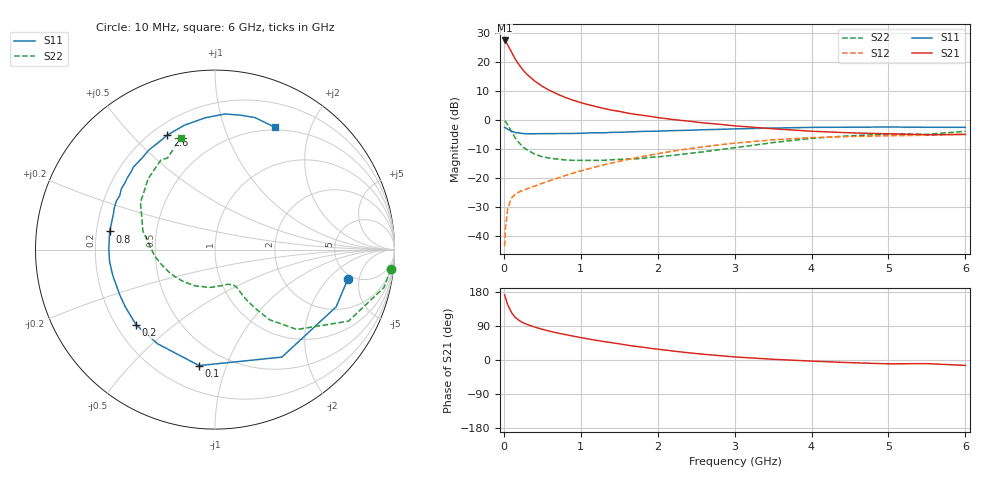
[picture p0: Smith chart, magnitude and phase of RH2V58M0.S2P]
! SIEMENS Small Signal Semiconductors
! BFR106
! Si NPN RF Bipolar Junction Transistor in SOT23
! VCE = 2.5 V  IC = 8 mA
! Common Emitter S-Parameters:  August  1996
# GHz  S  MA  R  50
!  f  S11  S21  S12  S22
! GHz  MAG  ANG  MAG  ANG  MAG  ANG  MAG  ANG
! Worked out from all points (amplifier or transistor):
!   36 points, 10 MHz to 6 GHz, reference 50 ohm
!   highest |S21| = 27.5 dB at 10 MHz (marker M1)
!   |S21| within 3 dB of that: start of sweep to 79.89 MHz
!   unconditionally stable (mu >= 1): 520.5 MHz to 2.169 GHz; 4.701 GHz to end of sweep
!   at 250 MHz: K = 0.65, MSG = 20.7 dB, |S12| = -24.1 dB
!   at 1.4 GHz: K = 1.12, MAG = 7.1 dB, |S12| = -14.7 dB
!   at 6 GHz: K = 1.02, MAG = -0.9 dB, |S12| = -4.7 dB
!   S11 on the Smith chart (normalised r, x): 10 MHz: 4.45, -3.48; 100 MHz: 0.36, -0.81; 200 MHz: 0.28, -0.37; 800 MHz: 0.26, +0.08; 2.6 GHz: 0.26, +0.64; 6 GHz: 0.47, +1.50
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0.01  0.7576 -12.7  23.84 171.8  0.0068 85.5  0.9853 -6.4
0.02  0.7465 -25.3  23.16 165.1  0.0136 77.2  0.9645 -12.7
0.05  0.7055 -58.1  20.09 145.8  0.03 62.7  0.8438 -28.2
0.1  0.6522 -97.8  15.01 125.1  0.0461 50.1  0.6373 -44.3
0.15  0.6146 -121.4  11.28 112.2  0.0535 43.5  0.4956 -52.1
0.2  0.6074 -136.3  9.002 104.3  0.0585 42.2  0.4084 -55.1
0.25  0.5934 -147.0  7.36 98.1  0.0623 42.5  0.3467 -57.4
0.3  0.5877 -154.5  6.226 93.9  0.066 43.7  0.3111 -58.5
0.4  0.5875 -165.8  4.782 87.0  0.0738 46.1  0.2628 -59.5
0.5  0.5911 -173.4  3.861 81.1  0.0823 49.3  0.236 -60.5
0.6  0.5916 180.0  3.257 75.8  0.0918 51.8  0.2233 -62.7
0.8  0.5956 170.2  2.483 67.0  0.1122 55.6  0.2077 -68.4
0.9  0.5953 165.8  2.225 63.0  0.1234 56.7  0.2048 -71.2
1.1  0.6074 157.4  1.863 55.5  0.1464 58.2  0.2047 -79.9
1.3  0.61 150.4  1.605 48.8  0.1714 58.5  0.2052 -88.5
1.6  0.6306 141.0  1.341 39.4  0.2106 57.6  0.2152 -103.1
2.2  0.6661 123.6  1.034 23.7  0.2954 51.8  0.2499 -134.1
2.6  0.6908 112.6  0.904 15.1  0.3517 46.1  0.2877 -155.0
3.5  0.737 94.0  0.717 1.9  0.4629 30.9  0.4145 165.6
4.5  0.7628 79.0  0.611 -7.0  0.5272 13.7  0.5429 133.3
5.5  0.7606 67.9  0.566 -9.6  0.5546 3.0  0.575 117.4
6  0.7589 64.0  0.572 -14.3  0.58 -4.5  0.649 107.2
